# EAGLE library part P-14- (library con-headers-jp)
HEADER PLUG PINS
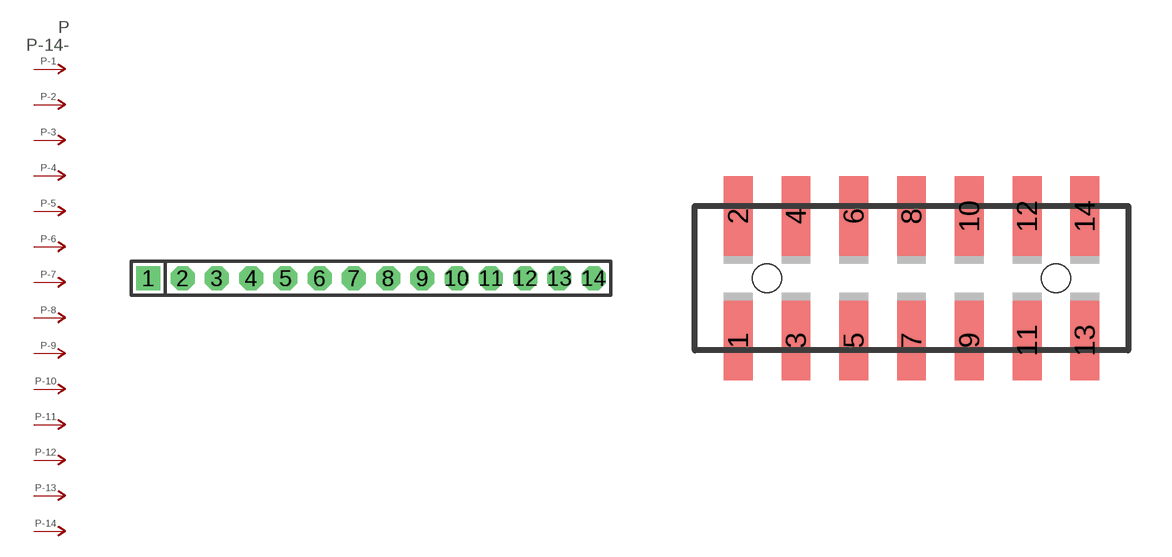
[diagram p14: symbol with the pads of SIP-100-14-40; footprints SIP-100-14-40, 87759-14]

Designator prefix P; gates -2=P-N -3=P-N -4=P-N -5=P-N -6=P-N -7=P-N -8=P-N -9=P-N -10=P-N -11=P-N -12=P-N -13=P-N -14=P-N -1=P-NV

## P-14-SIP-100-40  [SIP-100-14-40]
1  -1:P  pas
2  -2:P  pas
3  -3:P  pas
4  -4:P  pas
5  -5:P  pas
6  -6:P  pas
7  -7:P  pas
8  -8:P  pas
9  -9:P  pas
10  -10:P  pas
11  -11:P  pas
12  -12:P  pas
13  -13:P  pas
14  -14:P  pas

## P-14-87759  [87759-14]
Pads as for SIP-100-14-40

## P-14-100-2X07  [DIL-100-2X07]
Pads as for SIP-100-14-40

## P-14-100-2X07_M  [DIL-100-2X07_M]
Pads as for SIP-100-14-40

## P-14-2MM-2X07  [DIL-2MM-2X07]
Pads as for SIP-100-14-40

## P-14-2MM-2X07_M  [DIL-2MM-2X07_M]
Pads as for SIP-100-14-40

## P-14-SIP-100-32  [SIP-100-14-32]
Pads as for SIP-100-14-40

## P-14-SIP-100-40Y  [SIP-100-14-40Y]
Pads as for SIP-100-14-40

## P-14-SIP-100-32Y  [SIP-100-14-32Y]
Pads as for SIP-100-14-40

## P-14-87759_M  [87759-14_M]
Pads as for SIP-100-14-40

## P-14-LCW-114-XX-X-S  [LCW-114-XX-X-S]
Pads as for SIP-100-14-40

## P-14-LCW-114-XX-X-S-RE  [LCW-114-XX-X-S-RE]
Pads as for SIP-100-14-40

## Footprint SIP-100-14-40 (pad centres in mm)
SIP Header - 0.1", 40 mil drill
drill 1.016 pad 1.778 square: 1 -16.51,0
drill 1.016 pad 1.778 octagon: 2 -13.97,0; 3 -11.43,0; 4 -8.89,0; 5 -6.35,0; 6 -3.81,0; 7 -1.27,0; 8 1.27,0; 9 3.81,0; 10 6.35,0; 11 8.89,0; 12 11.43,0; 13 13.97,0; 14 16.51,0

## Footprint 87759-14 (pad centres in mm)
Molex PCB Pin Headers 2.00mm (.079") Pitch Milli-Grid Header, Vertical SMD
smd 1 x 2.75: 1 -6,-2.15; 2 -6,2.15; 3 -4,-2.15; 4 -4,2.15; 5 -2,-2.15; 6 -2,2.15; 7 0,-2.15; 8 0,2.15; 9 2,-2.15; 10 2,2.15; 11 4,-2.15; 12 4,2.15; 13 6,-2.15; 14 6,2.15
hole 1 at -5,0
hole 1 at 5,0

## Footprint DIL-100-2X07 (pad centres in mm)
PIN HEADER - 0.1"
drill 1.016 square: 1 -7.62,-1.27
drill 1.016 octagon: 2 -7.62,1.27; 3 -5.08,-1.27; 4 -5.08,1.27; 5 -2.54,-1.27; 6 -2.54,1.27; 7 0,-1.27; 8 0,1.27; 9 2.54,-1.27; 10 2.54,1.27; 11 5.08,-1.27; 12 5.08,1.27; 13 7.62,-1.27; 14 7.62,1.27

## Footprint DIL-100-2X07_M (pad centres in mm)
PIN HEADER - MIRRORED 0.1"
drill 1.016 square: 1 -7.62,1.27
drill 1.016 octagon: 2 -7.62,-1.27; 3 -5.08,1.27; 4 -5.08,-1.27; 5 -2.54,1.27; 6 -2.54,-1.27; 7 0,1.27; 8 0,-1.27; 9 2.54,1.27; 10 2.54,-1.27; 11 5.08,1.27; 12 5.08,-1.27; 13 7.62,1.27; 14 7.62,-1.27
